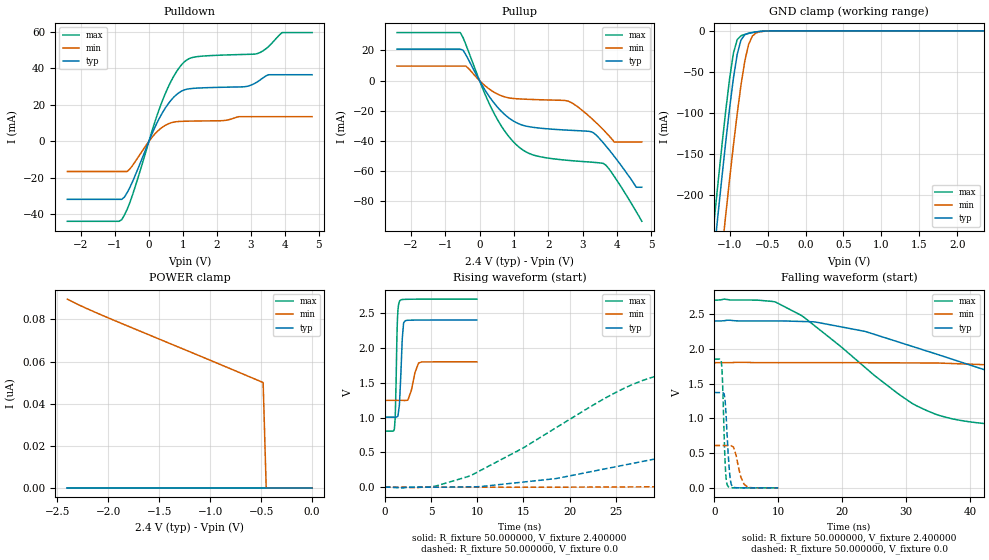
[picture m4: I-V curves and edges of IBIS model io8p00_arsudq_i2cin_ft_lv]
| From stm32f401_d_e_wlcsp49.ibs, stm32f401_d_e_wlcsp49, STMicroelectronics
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|   Model io8p00_arsudq_i2cin_ft_lv
[Model]  io8p00_arsudq_i2cin_ft_lv
Model_type I/O
Polarity   Non-Inverting
Enable   Active-Low
Vinl =   0.720000V
Vinh =   1.680000V
Vmeas =  1.200000V
Cref =   50.000000pF
Rref =   100.000000M
Vref =   0.0V
C_comp   2.226900pF   2.174000pF   2.332300pF
[Temperature Range]   25.000000   0.125000k   -40.000000
[Pullup Reference]   2.400000V   1.800000V   2.700000V
[Pulldown Reference]   0.0V   0.0V   0.0V
[POWER Clamp Reference]   2.400000V   1.800000V   2.700000V
[GND Clamp Reference]   0.0V   0.0V   0.0V
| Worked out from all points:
|   slope of the pulldown table from 0 to 0.36 V, typ, clamps not added: 25 ohm
|   slope of the pullup table from 0 to 0.36 V, typ, clamps not added: 27.7 ohm
|   GND clamp passes 1 mA (typ) near -0.62 V on its own axis
|   rising waveform, R_fixture 50.000000, V_fixture 2.400000: 20-80 % time 271ps typ, 605ps min, 184ps max; typ from 1.01 V to 2.4 V
|   rising waveform, R_fixture 50.000000, V_fixture 0.0: 20-80 % time 32.4ns typ, 81.1ns min, 14.7ns max; typ from 0 V to 1.37 V
|   falling waveform, R_fixture 50.000000, V_fixture 2.400000: 20-80 % time 29.2ns typ, 72ns min, 15.7ns max; typ from 2.4 V to 1.01 V
|   falling waveform, R_fixture 50.000000, V_fixture 0.0: 20-80 % time 523ps typ, 973ps min, 382ps max; typ from 1.37 V to 0 V
[Pulldown]
|Voltage   I(typ)   I(min)   I(max)
-2.4V     -31.73mA   -16.51mA   -43.74mA
-800mV    -31.73mA   -16.51mA   -42.87mA
-480mV    -21.98mA   -13.17mA   -29.21mA
80mV      3.63mA     1.966mA    5.014mA
480mV     18.16mA    8.738mA    26.02mA
800mV     25.38mA    10.72mA    37.77mA
1.12V     28.53mA    11.02mA    44.6mA
2.8V      29.84mA    13.49mA    47.53mA
3.2V      32.65mA    13.49mA    48.05mA
3.52V     36.43mA    13.49mA    51.84mA
3.92V     36.43mA    13.49mA    59.49mA
4.8V      36.43mA    13.49mA    59.49mA
[Pullup]
|Voltage   I(typ)   I(min)   I(max)
-2.4V     20.89mA    9.66mA     31.9mA
-560mV    20.89mA    9.66mA     31.9mA
-400mV    17.28mA    9.66mA     24.07mA
320mV     -11.75mA   -6.207mA   -17.08mA
960mV     -26.47mA   -11.82mA   -40.02mA
1.52V     -30.88mA   -12.51mA   -49.05mA
2.56V     -32.88mA   -13.48mA   -52.9mA
3.28V     -34.19mA   -25.52mA   -54.18mA
3.6V      -41.31mA   -32.61mA   -54.97mA
3.92V     -50.33mA   -40.8mA    -63.62mA
4.56V     -70.8mA    -40.8mA    -87.08mA
4.72V     -70.8mA    -40.8mA    -93.4mA
[GND_clamp]
|Voltage   I(typ)   I(min)   I(max)
-2.4V     -1.425A    -1.509A    -1.394A
-1.25V    -311.2mA   -401.9mA   -273.3mA
-1.2V     -265.4mA   -356.1mA   -227.2mA
-1.15V    -220.4mA   -310.8mA   -181.9mA
-1.1V     -176.3mA   -266.2mA   -137.9mA
-1.05V    -133.8mA   -222.5mA   -95.87mA
-950mV    -57.3mA    -138.9mA   -26.98mA
-900mV    -28.27mA   -100.4mA   -10.59mA
-850mV    -11.01mA   -65.54mA   -5.958mA
-750mV    -2.834mA   -16.5mA    -3.178mA
-600mV    -750uA     -1.164mA   -738.3uA
2.35V     0A         0A         0A
[POWER_clamp]
|Voltage   I(typ)   I(min)   I(max)
-2.4V     0A         89.62nA    0A
-2.04V    0A         81.57nA    0A
-480mV    0A         50.01nA    0A
-450mV    0A         0A         0A
0V        0A         0A         0A
[Ramp]
| variable   typ   min   max
dV/dt_r  0.82230/32.34958n   0.36200/82.85000n   1.11114/14.71607n
dV/dt_f  0.83784/29.25364n   0.32706/74.33462n   1.13768/15.72290n
R_load = 50.000000
[Rising Waveform]
R_fixture= 50.000000
V_fixture= 2.400000
V_fixture_min= 1.800000
V_fixture_max= 2.700000
|time   V(typ)   V(min)   V(max)
0s        1.006V     1.247V     804.6mV
1.041ns   1.006V     1.247V     839.1mV
1.141ns   1.006V     1.247V     1.059V
1.381ns   1.015V     1.247V     2.443V
1.642ns   1.343V     1.247V     2.678V
1.902ns   2.146V     1.247V     2.694V
2.162ns   2.384V     1.245V     2.697V
2.503ns   2.397V     1.252V     2.698V
3.664ns   2.399V     1.784V     2.699V
9.97ns    2.4V       1.8V       2.7V
[Rising Waveform]
R_fixture= 50.000000
V_fixture= 0.0
V_fixture_min= 0.0
V_fixture_max= 0.0
|time   V(typ)   V(min)   V(max)
0s        10.23nV    261.2nV    17.67nV
5.005ns   -211.5uV   -67.94uV   7.505mV
9.009ns   4.968mV    -58.81uV   153.1mV
18.52ns   123.8mV    457uV      852.2mV
28.53ns   386.5mV    5.785mV    1.56V
40.54ns   733.6mV    34.29mV    1.781V
65.57ns   1.237V     122mV      1.843V
79.08ns   1.314V     189.2mV    1.849V
148.1ns   1.368V     492.9mV    1.852V
249.2ns   1.37V      609.1mV    1.852V
[Falling Waveform]
R_fixture= 50.000000
V_fixture= 2.400000
V_fixture_min= 1.800000
V_fixture_max= 2.700000
|time   V(typ)   V(min)   V(max)
0s        2.4V       1.8V       2.7V
9.51ns    2.4V       1.8V       2.673V
16.02ns   2.381V     1.8V       2.305V
31.03ns   2.031V     1.796V     1.208V
36.54ns   1.869V     1.79V      1.006V
44.54ns   1.629V     1.763V     905.1mV
59.06ns   1.255V     1.715V     847.6mV
87.09ns   1.073V     1.558V     814.8mV
137.1ns   1.02V      1.353V     805.4mV
249.2ns   1.006V     1.247V     804.6mV
[Falling Waveform]
R_fixture= 50.000000
V_fixture= 0.0
V_fixture_min= 0.0
V_fixture_max= 0.0
|time   V(typ)   V(min)   V(max)
0s        1.37V      609.1mV    1.852V
1.061ns   1.37V      609.1mV    1.82V
1.261ns   1.37V      609mV      1.521V
1.662ns   1.255V     608.8mV    359.5mV
1.842ns   998.4mV    608.5mV    113.2mV
2.062ns   617.4mV    608.4mV    30.28mV
2.482ns   116.5mV    610.6mV    3.878mV
2.843ns   17.79mV    593.4mV    1.617mV
4.645ns   446.7uV    51.19mV    344.7uV
9.97ns    10.23nV    261.2nV    17.67nV
